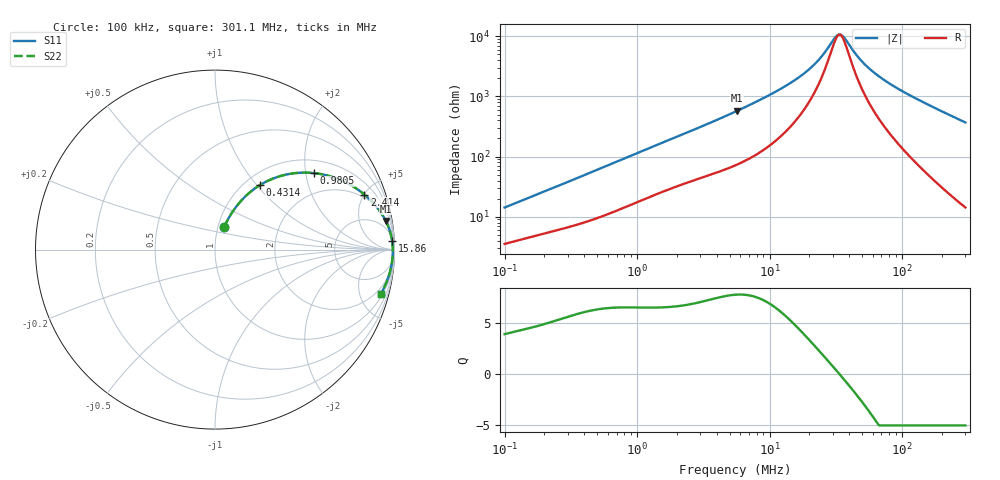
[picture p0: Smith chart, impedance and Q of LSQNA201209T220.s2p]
! LSQNA201209T220  S-PARAMETER MODEL  ( General Type )
! Model Generated by TAIYO YUDEN Corporation (http://www.ty-top.com)
! Version 2.0
! TAIYO YUDEN Control No. 100810NF25SB-FAC
! Copyright(c) 2007 TAIYO YUDEN CO.,LTD. All Rights Reserved.
! Product Description (link to TY-COMPAS)
! https://ds.yuden.co.jp/TYCOMPAS/or/detail?pn=LSQNA201209T220M&u=M
! Products Name : Inductors
! Characteristics :
!  Inductance : 22 uH , SRF(min) : 23 MHz , DC Resistance(max) : 2.73 Ohm
!  Rated Current : Saturation :150 mA , Temp Rise : 250 mA (40 degC)
!  Case Size : 2.0 x 1.25 / 0.079 x 0.049 [mm/inch] , Thickness : 0.9 / 0.035 [mm/inch]
!  (Conditions: Temperature = 25 degC , DC Bias Current/Voltage = 0A / 0V)
! External Node Assignments :
!  1  o---GGG---o  2
! GND o---------o GND
! Frequency Range : 0.1MHz  -  301.082333MHz  [ 402 STEP ]
# MHz S RI R 50
! Freq[MHz].  S11 Real  S11 Imag  S21 Real  S21 Imag  S12 Real  S12 Imag  S22 Real  S22 Imag
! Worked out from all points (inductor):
!   401 points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, 100 kHz to 301.1 MHz, reference 50 ohm
!   read as one part in series: L = 21.4 uH near 104.1 kHz
!   highest Q = 7.75 at 5.711 MHz (marker M1), where L = 16 uH
!   self-resonance near 33.27 MHz
!   S11 on the Smith chart (normalised r, x): 100 kHz: 1.07, +0.28; 431.4 kHz: 1.17, +1.04; 980.5 kHz: 1.34, +2.22; 2.414 MHz: 1.74, +5.02; 15.86 MHz: 9, +38; 301.1 MHz: 1.29, -7.38
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0.1  0.0509 0.1263  0.9491 -0.1263  0.9491 -0.1263  0.0509 0.1263
0.21403  0.1117 0.2304  0.8883 -0.2304  0.8883 -0.2304  0.1117 0.2304
0.382543  0.2186 0.3381  0.7814 -0.3381  0.7814 -0.3381  0.2186 0.3381
0.43138  0.2512 0.3599  0.7488 -0.3599  0.7488 -0.3599  0.2512 0.3599
0.670174  0.4012 0.419  0.5988 -0.419  0.5988 -0.419  0.4012 0.419
0.98045  0.5507 0.4264  0.4493 -0.4264  0.4493 -0.4264  0.5507 0.4264
1.463388  0.6961 0.3893  0.3039 -0.3893  0.3039 -0.3893  0.6961 0.3893
2.414223  0.8325 0.3068  0.1675 -0.3068  0.1675 -0.3068  0.8325 0.3068
5.487097  0.9484 0.1658  0.0516 -0.1658  0.0516 -0.1658  0.9484 0.1658
5.711314  0.9514 0.1599  0.0486 -0.1599  0.0486 -0.1599  0.9514 0.1599
10.208  0.9787 0.0884  0.0213 -0.0884  0.0213 -0.0884  0.9787 0.0884
15.85873  0.9868 0.0496  0.0132 -0.0496  0.0132 -0.0496  0.9868 0.0496
20.99048  0.9892 0.0296  0.0108 -0.0296  0.0108 -0.0296  0.9892 0.0296
25.13581  0.9901 0.018  0.00992 -0.018  0.00992 -0.018  0.9901 0.018
31.32973  0.9907 0.0045  0.00934 -0.0045  0.00934 -0.0045  0.9907 0.0045
33.94248  0.9907 -0.000332  0.00925 0.000332  0.00925 0.000332  0.9907 -0.000332
36.77311  0.9908 -0.00517  0.00922 0.00517  0.00922 0.00517  0.9908 -0.00517
44.92598  0.9906 -0.0175  0.00939 0.0175  0.00939 0.0175  0.9906 -0.0175
52.73163  0.9902 -0.0278  0.00981 0.0278  0.00981 0.0278  0.9902 -0.0278
80.29753  0.9875 -0.0589  0.0125 0.0589  0.0125 0.0589  0.9875 -0.0589
143.5182  0.9762 -0.1194  0.0238 0.1194  0.0238 0.1194  0.9762 -0.1194
301.0823  0.9233 -0.2474  0.0767 0.2474  0.0767 0.2474  0.9233 -0.2474
